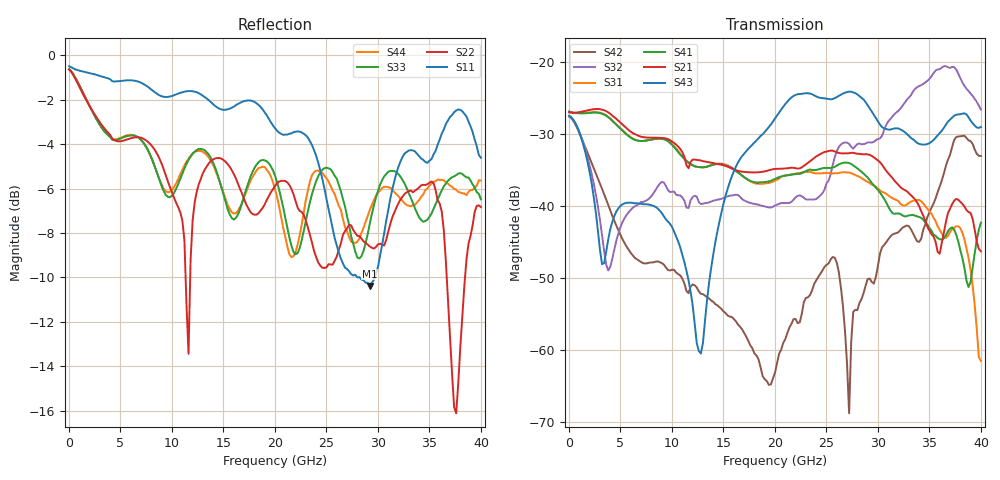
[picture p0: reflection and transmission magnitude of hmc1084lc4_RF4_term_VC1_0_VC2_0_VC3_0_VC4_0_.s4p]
!Agilent Technologies,N5224A,MY51441122,A.09.40.06
!Agilent N5224A: A.09.40.06
!Date: Thursday, June 19, 2014 00:53:39
!Correction: S11(Full 4 Port(1,2,3,4))
!S12(Full 4 Port(1,2,3,4))
!S13(Full 4 Port(1,2,3,4))
!S14(Full 4 Port(1,2,3,4))
!S21(Full 4 Port(1,2,3,4))
!S22(Full 4 Port(1,2,3,4))
!S23(Full 4 Port(1,2,3,4))
!S24(Full 4 Port(1,2,3,4))
!S31(Full 4 Port(1,2,3,4))
!S32(Full 4 Port(1,2,3,4))
!S33(Full 4 Port(1,2,3,4))
!S34(Full 4 Port(1,2,3,4))
!S41(Full 4 Port(1,2,3,4))
!S42(Full 4 Port(1,2,3,4))
!S43(Full 4 Port(1,2,3,4))
!S44(Full 4 Port(1,2,3,4))
!S4P File: Measurements: <S11,S12,S13,S14>,
!<S21,S22,S23,S24>,
!<S31,S32,S33,S34>,
!<S41,S42,S43,S44>:
# Hz S  dB  R 50
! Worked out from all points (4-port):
!   201 points, 10 MHz to 40 GHz, reference 50 ohm
!   strongest paths, dB at 10 MHz, 10.01 GHz, 20 GHz, 30 GHz, 40 GHz:
!     S43: -27.4, -42.9, -27.8, -28.2, -29.0
!     S21: -27.0, -31.0, -34.8, -33.7, -46.3
!     S41: -26.9, -31.5, -36.2, -37.8, -42.3
!     S31: -26.9, -31.4, -36.5, -37.6, -61.6
!     S32: -27.5, -38.0, -39.9, -30.7, -26.6
!     S42: -27.6, -48.9, -63.2, -48.3, -33.0
!   lowest |S11| = -10.4 dB at 29.2 GHz (marker M1), VSWR 1.87, Z = 77.8 + j28.2 ohm
!   |S11| at or under -10 dB: 28.00158 GHz to 28.01912 GHz (17.54 MHz wide, 0.0626 % of centre); 28.22 GHz to 29.68 GHz (1.465 GHz wide, 5.06 % of centre)
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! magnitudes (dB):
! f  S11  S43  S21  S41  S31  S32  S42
! 10 MHz  -0.5  -27.4  -27.0  -26.9  -26.9  -27.5  -27.6
! 3.809 GHz  -1.0  -44.6  -27.0  -27.6  -27.6  -49.0  -39.9
! 12.81 GHz  -1.8  -60.5  -33.7  -34.6  -34.6  -39.7  -52.2
! 16.81 GHz  -2.1  -33.1  -35.2  -35.8  -35.7  -39.0  -57.2
! 27.2 GHz  -9.7  -24.1  -32.7  -34.0  -35.4  -31.4  -68.8
! 29.2 GHz  -10.4  -26.4  -32.9  -36.4  -36.8  -31.1  -50.1
! 40 GHz  -4.6  -29.0  -46.3  -42.3  -61.6  -26.6  -33.0
